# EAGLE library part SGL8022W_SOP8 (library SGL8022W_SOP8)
Single-channel DC LED control touch chip Version 1.6 Source: Datasheet
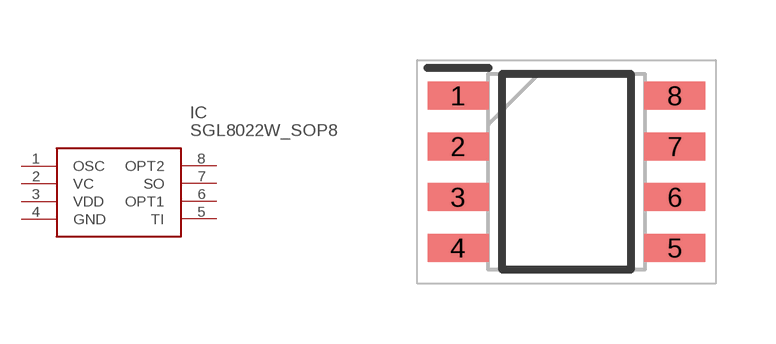
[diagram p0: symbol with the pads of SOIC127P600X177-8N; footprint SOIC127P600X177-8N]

Designator prefix IC

## SGL8022W_SOP8 (Description: Single-channel DC LED control touch chip Version 1.6; Height: 1.77mm; Manufacturer_Name: Sigma Designs Inc.; Manufacturer_Part_Number: SGL8022W/SOP8)  [SOIC127P600X177-8N]
1  OSC
2  VC
3  VDD
4  GND
5  TI
6  OPT1
7  SO
8  OPT2

## Footprint SOIC127P600X177-8N (pad centres in mm)
SOP8
smd 1.525 x 0.7: 1 -2.712,1.905; 2 -2.712,0.635; 3 -2.712,-0.635; 4 -2.712,-1.905; 5 2.712,-1.905; 6 2.712,-0.635; 7 2.712,0.635; 8 2.712,1.905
